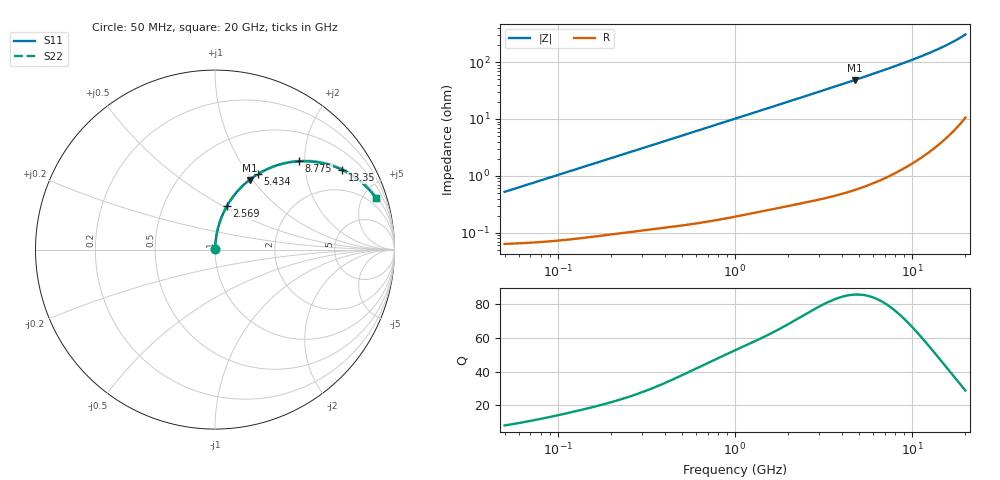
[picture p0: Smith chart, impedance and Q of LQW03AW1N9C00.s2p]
!Murata Part Number: LQW03AW1N9C00
!These Parameters are Measured in Series Mode Connection
!  o--[Z]--o
!Port1  Port2
!  o-------o
!Freq. Start=50[MHz] Stop=20[GHz], 401[Steps]
# Hz S RI R 50
!Freq.(Hz) S11(Real) S11(Imag) S21(Real) S21(Imag) S12(Real) S12(Imag) S22(Real) S22(Imag)
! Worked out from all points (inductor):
!   401 points, 50 MHz to 20 GHz, reference 50 ohm
!   read as one part in series: L = 1.65 nH near 51.52 MHz
!   highest Q = 85.7 at 4.748 GHz (marker M1), where L = 1.62 nH
!   S11 on the Smith chart (normalised r, x): 50 MHz: 1.00, +0.01; 2.569 GHz: 1.01, +0.52; 5.434 GHz: 1.01, +1.11; 8.775 GHz: 1.03, +1.88; 13.35 GHz: 1.06, +3.15; 20 GHz: 1.21, +6.10
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5e7  0.000664 0.00519  0.9993 -0.00519  0.9993 -0.00519  0.000664 0.00519
5.152053e7  0.000668 0.00535  0.9993 -0.00535  0.9993 -0.00535  0.000668 0.00535
1.364002e8  0.001 0.014  0.999 -0.014  0.999 -0.014  0.001 0.014
3.721004e8  0.00261 0.0377  0.9974 -0.0377  0.9974 -0.0377  0.00261 0.0377
6.285508e8  0.0055 0.0632  0.9945 -0.0632  0.9945 -0.0632  0.0055 0.0632
1e9  0.0119 0.0995  0.9881 -0.0995  0.9881 -0.0995  0.0119 0.0995
1.639343e9  0.0289 0.1598  0.9711 -0.1598  0.9711 -0.1598  0.0289 0.1598
2.569357e9  0.0656 0.2409  0.9344 -0.2409  0.9344 -0.2409  0.0656 0.2409
2.728004e9  0.0731 0.2538  0.9269 -0.2538  0.9269 -0.2538  0.0731 0.2538
3.626126e9  0.1215 0.3207  0.8785 -0.3207  0.8785 -0.3207  0.1215 0.3207
4.748272e9  0.1925 0.3885  0.8075 -0.3885  0.8075 -0.3885  0.1925 0.3885
5.433528e9  0.2393 0.4208  0.7607 -0.4208  0.7607 -0.4208  0.2393 0.4208
6.311513e9  0.3009 0.4527  0.6991 -0.4527  0.6991 -0.4527  0.3009 0.4527
7.442007e9  0.3799 0.4791  0.6201 -0.4791  0.6201 -0.4791  0.3799 0.4791
8.774992e9  0.4686 0.4922  0.5314 -0.4922  0.5314 -0.4922  0.4686 0.4922
9.745021e9  0.5285 0.4919  0.4715 -0.4919  0.4715 -0.4919  0.5285 0.4919
1.082228e10  0.5895 0.484  0.4105 -0.484  0.4105 -0.484  0.5895 0.484
1.201863e10  0.6501 0.4683  0.3499 -0.4683  0.3499 -0.4683  0.6501 0.4683
1.334722e10  0.7089 0.4447  0.2911 -0.4447  0.2911 -0.4447  0.7089 0.4447
1.621653e10  0.8084 0.3814  0.1916 -0.3814  0.1916 -0.3814  0.8084 0.3814
1.855685e10  0.8668 0.3249  0.1332 -0.3249  0.1332 -0.3249  0.8668 0.3249
2e10  0.8948 0.2899  0.1052 -0.2899  0.1052 -0.2899  0.8948 0.2899
